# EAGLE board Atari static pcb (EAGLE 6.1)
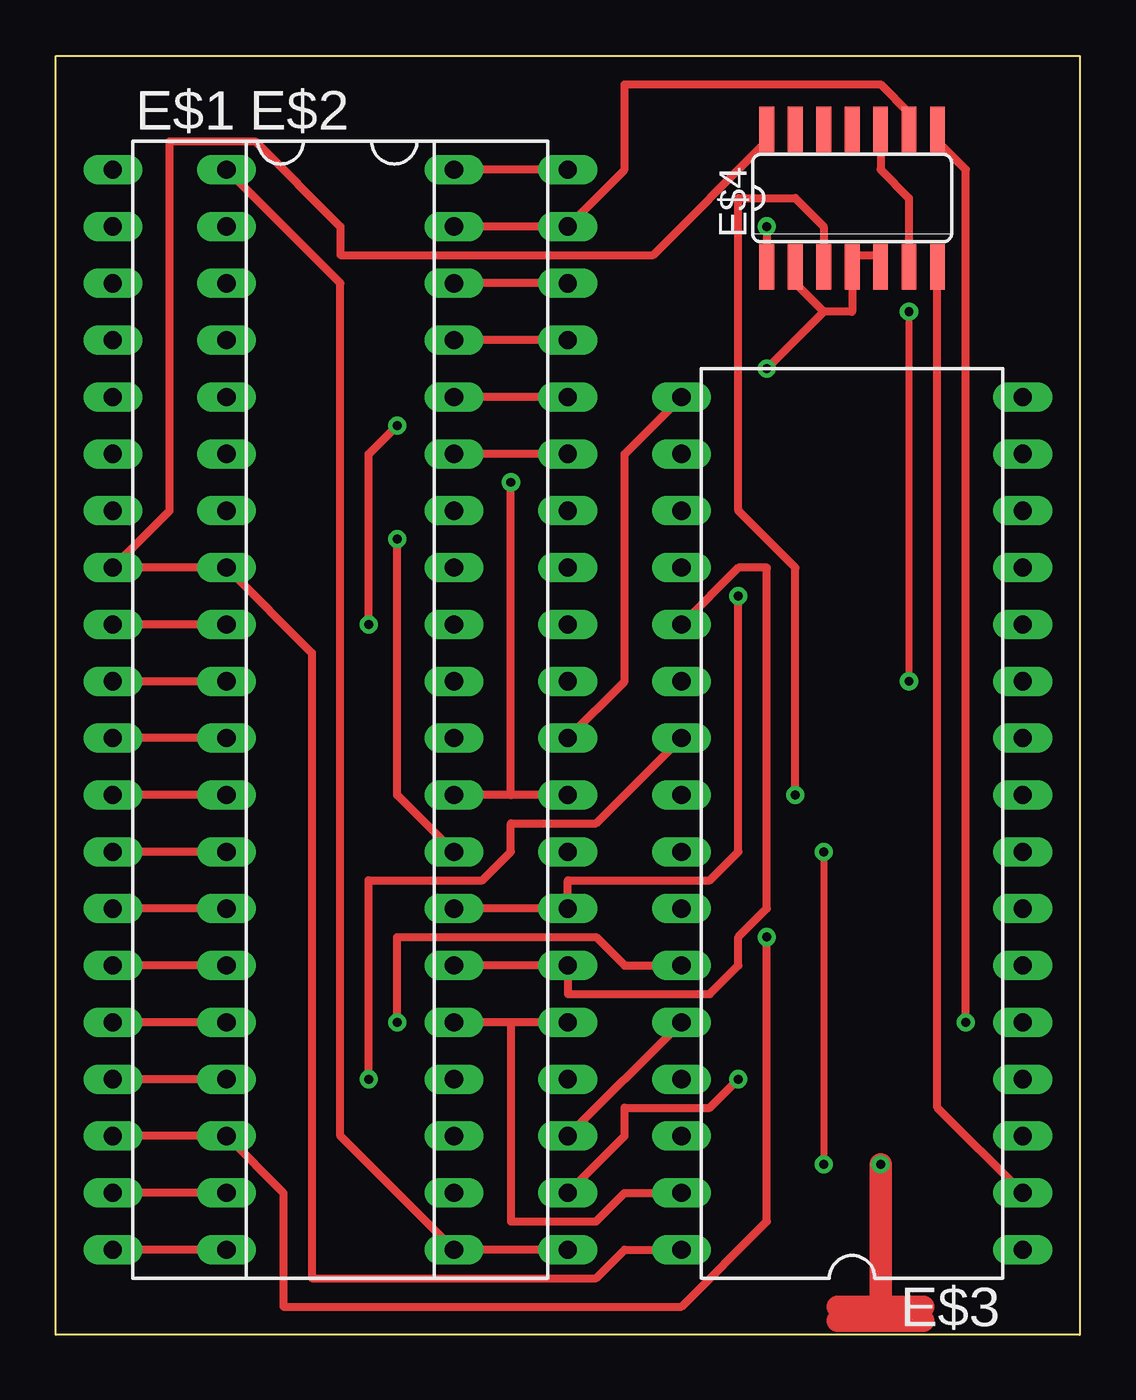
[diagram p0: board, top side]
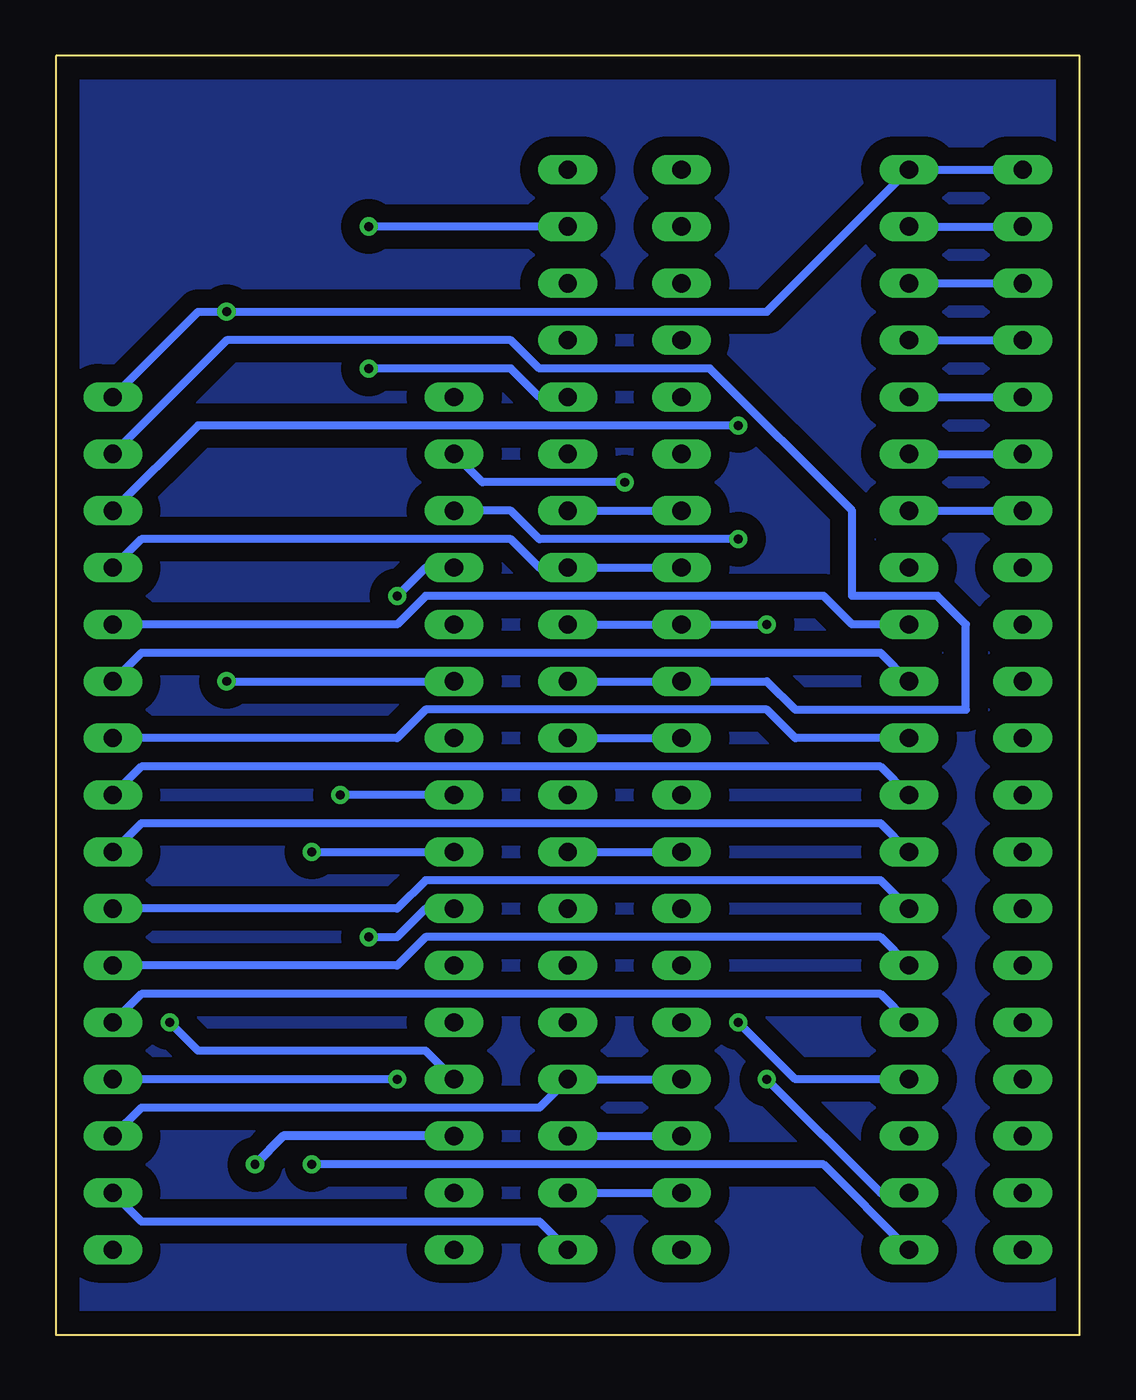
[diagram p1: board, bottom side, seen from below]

Size 45.72 x 57.15 mm. Coordinates in mm from the lower left corner, seen from the top.
Outline: 0,57.15 45.72,57.15 45.72,0 0,0 0,57.15
Copper layers (1*16): Top 0.035mm / dielectric 1.5mm / Bottom 0.035mm
Design rules: minimum track width 14mil, minimum drill 24mil, track to track 8mil, track to pad 8mil, pad to pad 8mil, via to via 8mil, smd to smd 8mil, copper to edge 40mil, drill to drill 8mil, minimum pad ring 10mil, minimum via ring 8mil, stop-mask expansion 4mil, vias tented up to drill 0mil, thermal gap 10mil

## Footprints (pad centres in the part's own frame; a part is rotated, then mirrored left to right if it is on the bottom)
DIL40 = drill 0.813 long: 1 -24.13,-7.62; 2 -21.59,-7.62; 3 -19.05,-7.62; 4 -16.51,-7.62; 5 -13.97,-7.62; 6 -11.43,-7.62; 7 -8.89,-7.62; 8 -6.35,-7.62; 9 -3.81,-7.62; 10 -1.27,-7.62; 11 1.27,-7.62; 12 3.81,-7.62; 13 6.35,-7.62; 14 8.89,-7.62; 15 11.43,-7.62; 16 13.97,-7.62; 17 16.51,-7.62; 18 19.05,-7.62; 19 21.59,-7.62; 20 24.13,-7.62; 21 24.13,7.62; 22 21.59,7.62; 23 19.05,7.62; 24 16.51,7.62; 25 13.97,7.62; 26 11.43,7.62; 27 8.89,7.62; 28 6.35,7.62; 29 3.81,7.62; 30 1.27,7.62; 31 -1.27,7.62; 32 -3.81,7.62; 33 -6.35,7.62; 34 -8.89,7.62; 35 -11.43,7.62; 36 -13.97,7.62; 37 -16.51,7.62; 38 -19.05,7.62; 39 -21.59,7.62; 40 -24.13,7.62
DIL32 = drill 0.813 long: 1 -19.05,-7.62; 2 -16.51,-7.62; 3 -13.97,-7.62; 4 -11.43,-7.62; 5 -8.89,-7.62; 6 -6.35,-7.62; 7 -3.81,-7.62; 8 -1.27,-7.62; 9 1.27,-7.62; 10 3.81,-7.62; 11 6.35,-7.62; 12 8.89,-7.62; 13 11.43,-7.62; 14 13.97,-7.62; 15 16.51,-7.62; 16 19.05,-7.62; 17 19.05,7.62; 18 16.51,7.62; 19 13.97,7.62; 20 11.43,7.62; 21 8.89,7.62; 22 6.35,7.62; 23 3.81,7.62; 24 1.27,7.62; 25 -1.27,7.62; 26 -3.81,7.62; 27 -6.35,7.62; 28 -8.89,7.62; 29 -11.43,7.62; 30 -13.97,7.62; 31 -16.51,7.62; 32 -19.05,7.62
SO14 = smd 0.66 x 2.032: 1 -3.81,-3.073; 2 -2.54,-3.073; 3 -1.27,-3.073; 4 0,-3.073; 5 1.27,-3.073; 6 2.54,-3.073; 7 3.81,-3.073; 8 3.81,3.073; 9 2.54,3.073; 10 1.27,3.073; 11 0,3.073; 12 -1.27,3.073; 13 -2.54,3.073; 14 -3.81,3.073

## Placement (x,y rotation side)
E$1  [DIL40]  10.16,27.94 270 top
E$2  [DIL40]  15.24,27.94 270 top
E$3  [DIL32]  35.56,22.86 90 top
E$4  [SO14]  35.56,50.8 0 top

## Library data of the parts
E$1-E$3 = ic-package
E$4 = 74xx-us

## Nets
S$1: E$3.25
S$2: E$1.2 E$2.2
S$3: E$1.3 E$2.3
S$4: E$1.4 E$2.4
S$5: E$1.5 E$2.5
S$6: E$1.6 E$2.6
S$7: E$1.7 E$2.7
S$8: E$1.8 E$2.8 E$3.32 E$4.14
S$9: E$1.9 E$2.9 E$3.12
S$10: E$1.10 E$2.10 E$3.11
S$11: E$1.11 E$2.11 E$3.10
S$12: E$1.12 E$2.12 E$3.9
S$13: E$1.13 E$2.13 E$3.8
S$14: E$1.14 E$2.14 E$3.7
S$15: E$1.15 E$2.15 E$3.6
S$16: E$1.16 E$2.16 E$3.5
S$17: E$3.27
S$18: E$1.18 E$2.18
S$19: E$3.23
S$20: E$1.20 E$2.20
S$21: E$1.40 E$2.40
S$22: E$1.39 E$2.39 E$4.9
S$23: E$1.38 E$2.38
S$24: E$1.37 E$2.37
S$25: E$3.22
S$26: E$1.35 E$2.35
S$27: E$1.34 E$2.34
S$28: E$1.33 E$2.33 E$3.13
S$29: E$3.14
S$30: E$1.31 E$2.31 E$3.15
S$31: E$1.30 E$2.30 E$3.17
S$32: E$1.29 E$2.29
S$33: E$1.28 E$2.28 E$3.19
S$34: E$1.27 E$2.27
S$35: E$1.26 E$2.26 E$3.21
S$36: E$1.25 E$2.25 E$3.31
S$37: E$1.24 E$2.24 E$3.3
S$38: E$1.23 E$2.23 E$3.28
S$39: E$1.22 E$2.22
S$40: E$1.1 E$1.21 E$2.1 E$2.21 E$3.2 E$3.16 E$4.7
S$41: E$1.36 E$2.36
S$42: E$4.6 E$4.10
S$43: E$4.8
S$44: E$4.3
S$45: E$1.32 E$2.32
S$46: E$1.17 E$2.17
S$47: E$1.19 E$2.19
S$48: E$3.18
S$49: E$4.1
S$50: E$4.2 E$4.4 E$4.5
S$53: E$3.20
S$54: E$3.24
S$55: E$3.26
S$56: E$3.29
S$57: E$3.4
S$73: E$3.30

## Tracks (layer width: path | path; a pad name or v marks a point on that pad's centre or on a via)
S$1
  Bottom 0.356: 34.29,21.59 E$3.25
S$2
  Bottom 0.356: E$2.2 E$1.2
S$3
  Bottom 0.356: E$2.3 E$1.3
S$4
  Bottom 0.356: E$2.4 E$1.4
S$5
  Bottom 0.356: E$2.5 E$1.5
S$6
  Bottom 0.356: E$2.6 E$1.6
S$7
  Bottom 0.356: E$2.7 E$1.7
S$8
  Top 0.356: E$4.14 31.75,53.34 26.67,48.26 12.7,48.26 12.7,49.53 8.89,53.34 5.08,53.34 5.08,36.83 E$1.8 E$2.8 11.43,30.48 11.43,2.54 24.13,2.54 25.4,3.81 E$3.32
S$9
  Top 0.356: E$2.9 E$1.9
  Bottom 0.356: E$3.12 30.48,31.75 29.21,33.02 11.43,33.02 10.16,31.75 E$2.9
S$10
  Top 0.356: E$2.10 E$1.10
  Bottom 0.356: E$3.11 41.91,30.48 8.89,30.48 E$2.10
S$11
  Top 0.356: E$2.11 E$1.11
  Bottom 0.356: E$3.10 30.48,26.67 29.21,27.94 13.97,27.94 12.7,26.67 E$2.11
S$12
  Top 0.356: E$2.12 E$1.12
  Bottom 0.356: E$3.9 41.91,25.4 8.89,25.4 E$2.12
S$13
  Top 0.356: E$2.13 E$1.13
  Bottom 0.356: E$3.8 41.91,22.86 8.89,22.86 E$2.13
S$14
  Top 0.356: E$2.14 E$1.14
  Bottom 0.356: E$3.7 30.48,19.05 29.21,20.32 8.89,20.32 E$2.14
S$15
  Top 0.356: E$2.15 E$1.15
  Bottom 0.356: E$3.6 30.48,16.51 29.21,17.78 8.89,17.78 E$2.15
S$16
  Top 0.356: E$2.16 E$1.16
  Bottom 0.356: E$3.5 41.91,15.24 8.89,15.24 E$2.16
S$17
  Top 0.356: E$3.27 25.4,16.51 24.13,17.78 15.24,17.78 15.24,13.97
S$18
  Top 0.356: E$1.18 E$2.18 10.16,6.35 10.16,1.27 27.94,1.27 31.75,5.08 31.75,17.78
S$19
  Top 0.356: E$3.23 24.13,22.86 20.32,22.86 20.32,21.59 19.05,20.32 13.97,20.32 13.97,11.43
S$20
  Top 0.356: E$2.20 E$1.20
  Bottom 0.356: 34.29,7.62 11.43,7.62 E$2.20
S$21
  Top 0.356: E$2.40 E$1.40
S$22
  Top 0.356: E$4.9 38.1,54.61 36.83,55.88 25.4,55.88 25.4,52.07 E$2.39 E$1.39
  Bottom 0.356: E$2.39 31.75,49.53
S$23
  Top 0.356: E$2.38 E$1.38
S$24
  Top 0.356: E$2.37 E$1.37
S$25
  Bottom 0.356: 38.1,29.21 E$3.22
S$26
  Top 0.356: E$2.35 E$1.35
S$27
  Bottom 0.356: E$2.34 E$1.34
S$28
  Bottom 0.356: E$1.33 E$2.33 24.13,34.29 25.4,35.56 41.91,35.56 E$3.13
S$29  (via drill 0.4 pad 0.81)
  Top 0.356: v15.24,40.64 13.97,39.37 13.97,31.75
  Bottom 0.356: E$3.14 39.37,40.64 v15.24,40.64
S$30
  Bottom 0.356: E$2.31 E$1.31 13.97,29.21 12.7,27.94 5.08,27.94 5.08,31.75 6.35,33.02 10.16,33.02 10.16,36.83 16.51,43.18 24.13,43.18 25.4,44.45 38.1,44.45 E$3.15
S$31
  Top 0.356: E$3.17 25.4,39.37 25.4,29.21 E$2.30
  Bottom 0.356: E$2.30 E$1.30
S$32
  Top 0.356: E$2.29 20.32,24.13 | 20.32,24.13 E$1.29 | 20.32,24.13 20.32,38.1
S$33  (via drill 0.4 pad 0.81)
  Top 0.356: v15.24,35.56 15.24,24.13 E$1.28
  Bottom 0.356: E$2.28 E$1.28 | E$3.19 25.4,36.83 24.13,35.56 v15.24,35.56
S$34
  Top 0.356: E$1.27 E$2.27 22.86,20.32 29.21,20.32 30.48,21.59 30.48,33.02
S$35
  Top 0.356: E$1.26 E$2.26 22.86,15.24 29.21,15.24 30.48,16.51 30.48,17.78 31.75,19.05 31.75,34.29 30.48,34.29 E$3.21
S$36
  Top 0.356: E$2.25 20.32,13.97 | 20.32,13.97 E$1.25 | E$3.31 25.4,6.35 24.13,5.08 20.32,5.08 20.32,13.97
S$37
  Bottom 0.356: E$1.24 E$2.24 24.13,10.16 41.91,10.16 E$3.3
S$38
  Top 0.356: E$2.23 E$3.28
  Bottom 0.356: E$2.23 E$1.23
S$39
  Top 0.356: 30.48,11.43 29.21,10.16 25.4,10.16 25.4,8.89 E$2.22
  Bottom 0.356: E$2.22 E$1.22
S$40
  Top 0.356: E$2.21 E$1.21 12.7,8.89 12.7,46.99 E$2.1 | E$4.7 39.37,10.16 E$3.2
  Bottom 0.356: E$1.1 E$2.1 13.97,45.72 39.37,45.72 E$3.16 | E$2.21 24.13,5.08 41.91,5.08 E$3.2
S$41
  Top 0.356: E$2.36 E$1.36
  Bottom 0.356: 31.75,43.18 25.4,43.18 24.13,41.91 E$2.36
S$42
  Top 0.356: E$4.6 38.1,50.8 36.83,52.07 E$4.10
S$43
  Top 0.356: 40.64,13.97 40.64,52.07 39.37,53.34 E$4.8
S$44
  Top 0.356: E$4.3 34.29,49.53 33.02,50.8 30.48,50.8 30.48,36.83 33.02,34.29 33.02,24.13
S$45
  Bottom 0.356: E$2.32 E$1.32 13.97,31.75
S$46
  Top 0.356: E$2.17 E$1.17
  Bottom 0.356: 15.24,13.97 12.7,11.43 E$2.17
S$47
  Top 0.356: E$2.19 E$1.19
  Bottom 0.356: 13.97,11.43 8.89,6.35 E$2.19
S$48
  Bottom 0.356: E$3.18 26.67,38.1 20.32,38.1
S$49
  Top 0.356: 31.75,49.53 E$4.1
S$50
  Top 0.356: E$4.5 36.83,48.26 35.56,48.26 E$4.4 35.56,45.72 34.29,45.72 | E$4.2 33.02,46.99 34.29,45.72 | 31.75,43.18 34.29,45.72
S$51
  Top 0.305: 34.29,21.59 34.29,7.62
S$52
  Top 0.305: 38.1,45.72 38.1,29.21
S$53
  Bottom 0.356: E$3.20 29.21,34.29 30.48,33.02
S$54
  Bottom 0.356: E$3.24 33.02,24.13
S$55
  Bottom 0.356: 31.75,17.78 30.48,17.78 29.21,19.05 E$3.26
S$56
  Bottom 0.356: 40.64,13.97 39.37,12.7 29.21,12.7 E$3.29
S$57
  Bottom 0.356: 30.48,11.43 E$3.4
S$58  (via drill 0.4 pad 0.81)
  other vias: 15.24,13.97
S$59  (via drill 0.4 pad 0.81)
  other vias: 13.97,11.43
S$60  (via drill 0.4 pad 0.81)
  other vias: 13.97,31.75
S$61  (via drill 0.4 pad 0.81)
  other vias: 20.32,38.1
S$62  (via drill 0.4 pad 0.81)
  other vias: 31.75,49.53
S$63  (via drill 0.4 pad 0.81)
  other vias: 31.75,43.18
S$64  (via drill 0.4 pad 0.81)
  other vias: 38.1,45.72
S$65  (via drill 0.4 pad 0.81)
  other vias: 40.64,13.97
S$66  (via drill 0.4 pad 0.81)
  other vias: 30.48,33.02
S$67  (via drill 0.4 pad 0.81)
  other vias: 38.1,29.21
S$68  (via drill 0.4 pad 0.81)
  other vias: 33.02,24.13
S$69  (via drill 0.4 pad 0.81)
  other vias: 34.29,21.59
S$70  (via drill 0.4 pad 0.81)
  other vias: 31.75,17.78
S$71  (via drill 0.4 pad 0.81)
  other vias: 30.48,11.43
S$72  (via drill 0.4 pad 0.81)
  Top 1.016: v36.83,7.62 36.83,0.63
S$73
  Bottom 0.406: E$3.30 35.56,8.89 36.83,7.62
S$74  (via drill 0.4 pad 0.81)
  other vias: 34.29,7.62
S$75
  Top 1.016: 34.93,0.63 35.56,0.63 | 38.74,0.63 35.56,0.63 | 35.56,0.63 34.93,1.27 38.74,1.27
S$76
  pour Bottom (isolate 0.813): 0,57.15 45.72,57.15 45.72,0 0,0

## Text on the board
tDocu: CAS Inhibit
